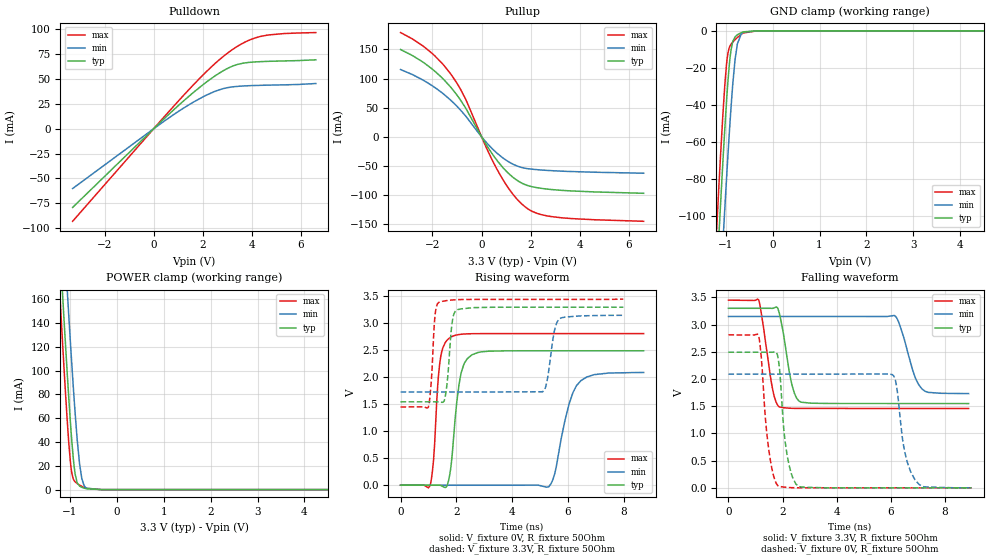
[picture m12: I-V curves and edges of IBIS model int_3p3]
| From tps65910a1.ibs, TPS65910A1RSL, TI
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|   int_3p3 Model
[Model]   int_3p3
Model_type   3-state
Polarity   Non-Inverting
Vmeas = 1.65
Vref = 0
Cref = 35pF
Rref = 50
|   typ   min   max
|   (nom PVT)   (fast PVT)   (slow PVT)
C_comp   1.060e-12   9.710e-13   1.280e-12
| Where nom  PVT is Nominal Process, 3.3V, 27C
|   Fast PVT is Strong Process,  3.45V, -40C
|   Slow PVT is Weak Process,   3.15V, 125C
[Voltage Range]   3.3   3.15   3.45
|Junction Temperature
[Temperature Range]   27   125   -40
[Pullup Reference]   3.3   3.15   3.45
[Pulldown Reference]   0   0   0
[Power Clamp Reference]   3.3   3.15   3.45
[GND Clamp Reference]   0   0   0
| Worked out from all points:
|   slope of the pulldown table from 0 to 0.495 V, typ, clamps not added: 42.3 ohm
|   slope of the pullup table from 0 to 0.495 V, typ, clamps not added: 15.1 ohm
|   GND clamp passes 1 mA (typ) near -0.67 V on its own axis
|   POWER clamp passes 1 mA (typ) near -0.67 V on its own axis
|   falling waveform, V_fixture 3.3V, R_fixture 50Ohm: 20-80 % time 356ps typ, 500ps min, 352ps max; typ from 3.3 V to 1.55 V
|   rising waveform, V_fixture 0V, R_fixture 50Ohm: 20-80 % time 300ps typ, 542ps min, 208ps max; typ from 0 V to 2.49 V
|   rising waveform, V_fixture 3.3V, R_fixture 50Ohm: 20-80 % time 165ps typ, 238ps min, 130ps max; typ from 1.55 V to 3.3 V
|   falling waveform, V_fixture 0V, R_fixture 50Ohm: 20-80 % time 288ps typ, 382ps min, 295ps max; typ from 2.49 V to 0 V
[Pulldown]
|   Voltage   I(typ)   I(min)   I(max)
-3.3V     -79.26mA   -60.23mA   -93.19mA
64.2mV    1.543mA    1.17mA     1.816mA
1.016V    23.6mA     17.59mA    28.19mA
2.072V    45.62mA    32.96mA    55.75mA
2.553V    54.15mA    38.21mA    66.93mA
2.934V    59.84mA    41.03mA    74.79mA
3.29V     63.84mA    42.42mA    81.15mA
3.635V    66.03mA    43.09mA    86.25mA
3.883V    66.84mA    43.39mA    89.2mA
4.34V     67.62mA    43.76mA    92.97mA
5.347V    68.36mA    44.28mA    95.96mA
6.6V      69.46mA    45.57mA    96.91mA
[GND Clamp]
|   Voltage   I(typ)   I(min)   I(max)
-3.3V     -1.256A    -1.281A    -1.245A
-1.25V    -162.6mA   -205.9mA   -136.1mA
-1.143V   -110mA     -154mA     -83.3mA
-1.119V   -98.2mA    -142.2mA   -71.63mA
-1.057V   -69.87mA   -113.6mA   -44.41mA
-1.02V    -53.49mA   -96.55mA   -29.82mA
-966.9mV  -32.63mA   -73.51mA   -14.73mA
-887.7mV  -10.6mA    -42.03mA   -7.289mA
-798.9mV  -3.249mA   -15.32mA   -4.773mA
-750.7mV  -2.146mA   -7.104mA   -3.623mA
-669.9mV  -1mA       -1.75mA    -1.945mA
6.6V      0A         0A         0A
[Pullup]
|   Voltage   I(typ)   I(min)   I(max)
-3.3V     149.8mA    115.5mA    178.9mA
-2.79V    138.8mA    106.3mA    167.3mA
-2.015V   116.5mA    87.84mA    143.2mA
-1.238V   84.18mA    62.07mA    106.7mA
-650.9mV  49.52mA    35.79mA    64.84mA
117.7mV   -8.47mA    -5.961mA   -11.45mA
656.7mV   -42.04mA   -29.12mA   -57.95mA
1.251V    -68.56mA   -46.38mA   -97.2mA
1.835V    -83.03mA   -54.42mA   -122.2mA
2.436V    -88.48mA   -56.99mA   -133.6mA
3.227V    -91.8mA    -58.9mA    -138.9mA
6.6V      -96.94mA   -62.5mA    -145mA
[POWER Clamp]
|   Voltage   I(typ)   I(min)   I(max)
-3.3V     1.818A     1.858A     1.815A
-1.295V   263.6mA    333.6mA    224.1mA
-1.171V   175.3mA    246.2mA    134.4mA
-1.145V   157.4mA    228.3mA    116.3mA
-1.063V   102.2mA    172.3mA    62.15mA
-978.1mV  51.32mA    117.7mA    19.66mA
-902.9mV  17.68mA    72.85mA    7.25mA
-841.5mV  5.613mA    41.27mA    5.044mA
-745.3mV  1.945mA    9.413mA    2.743mA
-644.5mV  739.3uA    1.186mA    1.023mA
-330.4mV  386.1nA    1.299uA    145.9nA
6.6V      0A         0A         0A
[Ramp]
R_load = 50
|   typ   min   max
dV/dt_r   1.49552/2.98967e-10   1.25422/5.38383e-10   1.68646/2.06808e-10
dV/dt_f   1.05027/3.54588e-10   0.850721/4.96374e-10   1.19254/3.50645e-10
[Falling Waveform]
V_fixture = 3.3V
V_fixture_min = 3.15V
V_fixture_max = 3.45V
R_fixture = 50Ohm
|   Time   V(typ)   V(min)   V(max)
0s        3.3V       3.15V      3.45V
1.114ns   3.3V       3.15V      3.458V
1.62ns    3.299V     3.15V      1.846V
1.88ns    3.212V     3.15V      1.489V
2.356ns   1.876V     3.15V      1.462V
2.694ns   1.574V     3.15V      1.46V
6.132ns   1.55V      3.167V     1.458V
6.878ns   1.55V      2.063V     1.458V
7.15ns    1.55V      1.821V     1.458V
8.88ns    1.55V      1.732V     1.457V
[Rising Waveform]
V_fixture = 0V
V_fixture_min = 0V
V_fixture_max = 0V
R_fixture = 50Ohm
|   Time   V(typ)   V(min)   V(max)
0s        628.9pV    1.216nV    571.2pV
1.056ns   -34.18nV   1.219nV    -13.17mV
1.186ns   3.8uV      1.212nV    479mV
1.41ns    684.8uV    1.211nV    2.27V
1.77ns    210.7mV    1.216nV    2.734V
2.138ns   1.988V     1.217nV    2.796V
2.554ns   2.416V     1.217nV    2.809V
5.318ns   2.492V     -27.73mV   2.811V
6.312ns   2.492V     1.847V     2.811V
8.721ns   2.493V     2.09V      2.811V
[Rising Waveform]
V_fixture = 3.3V
V_fixture_min = 3.15V
V_fixture_max = 3.45V
R_fixture = 50Ohm
|   Time   V(typ)   V(min)   V(max)
0s        1.546V     1.729V     1.451V
996ps     1.546V     1.729V     1.444V
1.236ns   1.546V     1.729V     3.141V
1.372ns   1.548V     1.729V     3.389V
1.588ns   1.597V     1.729V     3.417V
1.842ns   2.981V     1.729V     3.433V
2.05ns    3.255V     1.729V     3.44V
5.1ns     3.3V       1.733V     3.445V
5.682ns   3.3V       3.077V     3.445V
7.99ns    3.3V       3.15V      3.45V
[Falling Waveform]
V_fixture = 0V
V_fixture_min = 0V
V_fixture_max = 0V
R_fixture = 50Ohm
|   Time   V(typ)   V(min)   V(max)
0s        2.493V     2.09V      2.811V
1.11ns    2.493V     2.09V      2.803V
1.486ns   2.493V     2.09V      719.8mV
1.862ns   2.297V     2.09V      28.42mV
2.162ns   621.5mV    2.09V      8.446mV
2.618ns   21.41mV    2.09V      1.045mV
6.054ns   53.08uV    2.082V     41.04uV
6.522ns   47.43uV    653.4mV    35.71uV
6.894ns   43.4uV     151mV      32.03uV
8.99ns    3.105uV    7.112uV    1.227uV
